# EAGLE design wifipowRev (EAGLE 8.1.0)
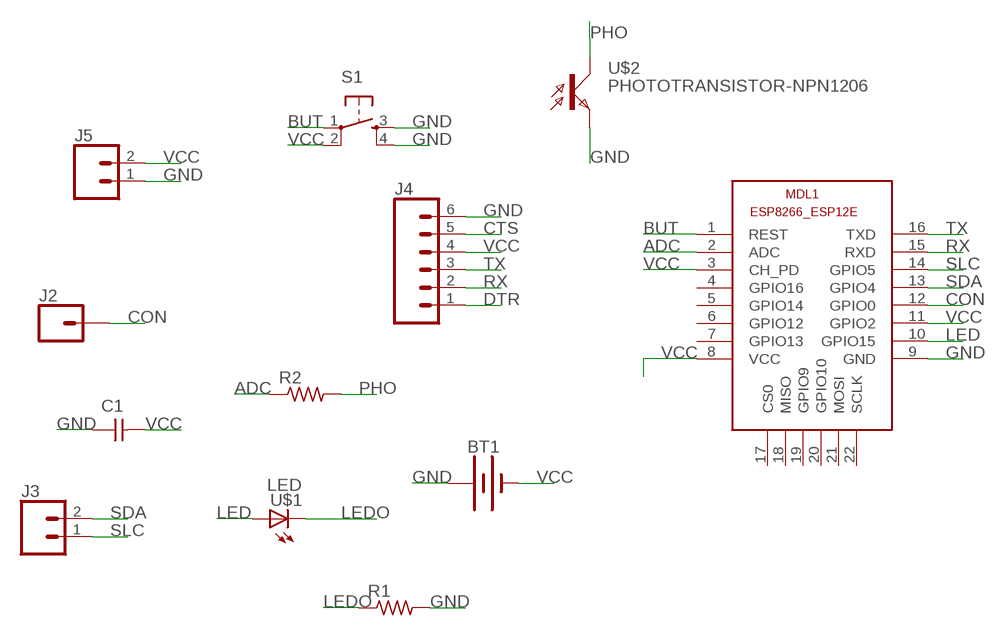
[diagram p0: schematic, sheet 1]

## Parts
BT1  BATTERY-20MM_SMD  [BATTCON_20MM]
C1  CAP-UNPOLARIZEDFAB  [C1206FAB]
J2  CONN_01PTH_LONGPAD  [1X01_LONGPAD]
J3  CONN_02PTH3  [1X02_LONGPADS]
J4  CONN_06LONGPADS  [1X06_LONGPADS]
J5  CONN_02PTH3  [1X02_LONGPADS]
MDL1  ESP8266-12EESP8266-ESP12E  [ESP8266-ESP12E]
R1  RES-US1206  [R1206]
R2  RES-US1206FAB  [R1206FAB]
S1  6MM_SWITCH6MM_SWITCH  [6MM_SWITCH]
U$1  LED  [LED1206]
U$2  PHOTOTRANSISTOR-NPN1206  [OP1206]

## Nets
ADC: MDL1.2(ADC) R2.1
BUT: MDL1.1(REST) S1.1(P)
CON: J2.1 MDL1.12(GPIO0)
CTS: J4.5
DTR: J4.1
GND: BT1.1(+) C1.1 J4.6 J5.1 MDL1.9(GND) R1.2 S1.3(S) S1.4(S1) U$2.EMITTER(E)
LED: MDL1.10(GPIO15) U$1.1(A)
LEDO: R1.1 U$1.2(C)
PHO: R2.2 U$2.COLLECTOR(C)
RX: J4.2 MDL1.15(RXD)
SDA: J3.2 MDL1.13(GPIO4)
SLC: J3.1 MDL1.14(GPIO5)
TX: J4.3 MDL1.16(TXD)
VCC: BT1.2(-) C1.2 J4.4 J5.2 MDL1.3(CH_PD) MDL1.8(VCC) MDL1.11(GPIO2) S1.2(P1)
Unconnected: MDL1.4(GPIO16) MDL1.5(GPIO14) MDL1.6(GPIO12) MDL1.7(GPIO13) MDL1.17(CS0) MDL1.18(MISO) MDL1.19(GPIO9) MDL1.20(GPIO10) MDL1.21(MOSI) MDL1.22(SCLK)

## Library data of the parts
BT1 = SparkFun-Batteries:BATTERY: Battery - Single Cell; PROD_ID: BATT-11519
C1 = fab:CAP-UNPOLARIZED
J2 = SparkFun-Connectors:CONN_01: Single connection point. Often used as Generic Header-pin footprint for 0.1 inch spaced/style header connections
J3 J5 = SparkFun-Connectors:CONN_02: Multi connection point. Often used as Generic Header-pin footprint for 0.1 inch spaced/style header connections
J4 = SparkFun-Connectors:CONN_06: Multi connection point. Often used as Generic Header-pin footprint for 0.1 inch spaced/style header connections On any of the 0.1 inch spaced packages, you can populate with these: Break Away Headers - Straight (PRT-00116) Break Away Male Headers - Right Angle (PRT-00553) Female Headers (PRT-00115)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
MDL1 = ESP8266-ESP12E:ESP8266-12E: ESP8266-12E with additional I/O and GPIO04/05 corrected The author cannot warrant that this library is free from error or will meet your specific requirements. Created by PuceBaboon.com. Komagane, Nagano, JAPAN
R1 R2 = fab:RES-US: Resistor (US Symbol)
S1 = fab:6MM_SWITCH: OMRON SWITCH
U$1 = fab:LED: LED
U$2 = fab:PHOTOTRANSISTOR-NPN

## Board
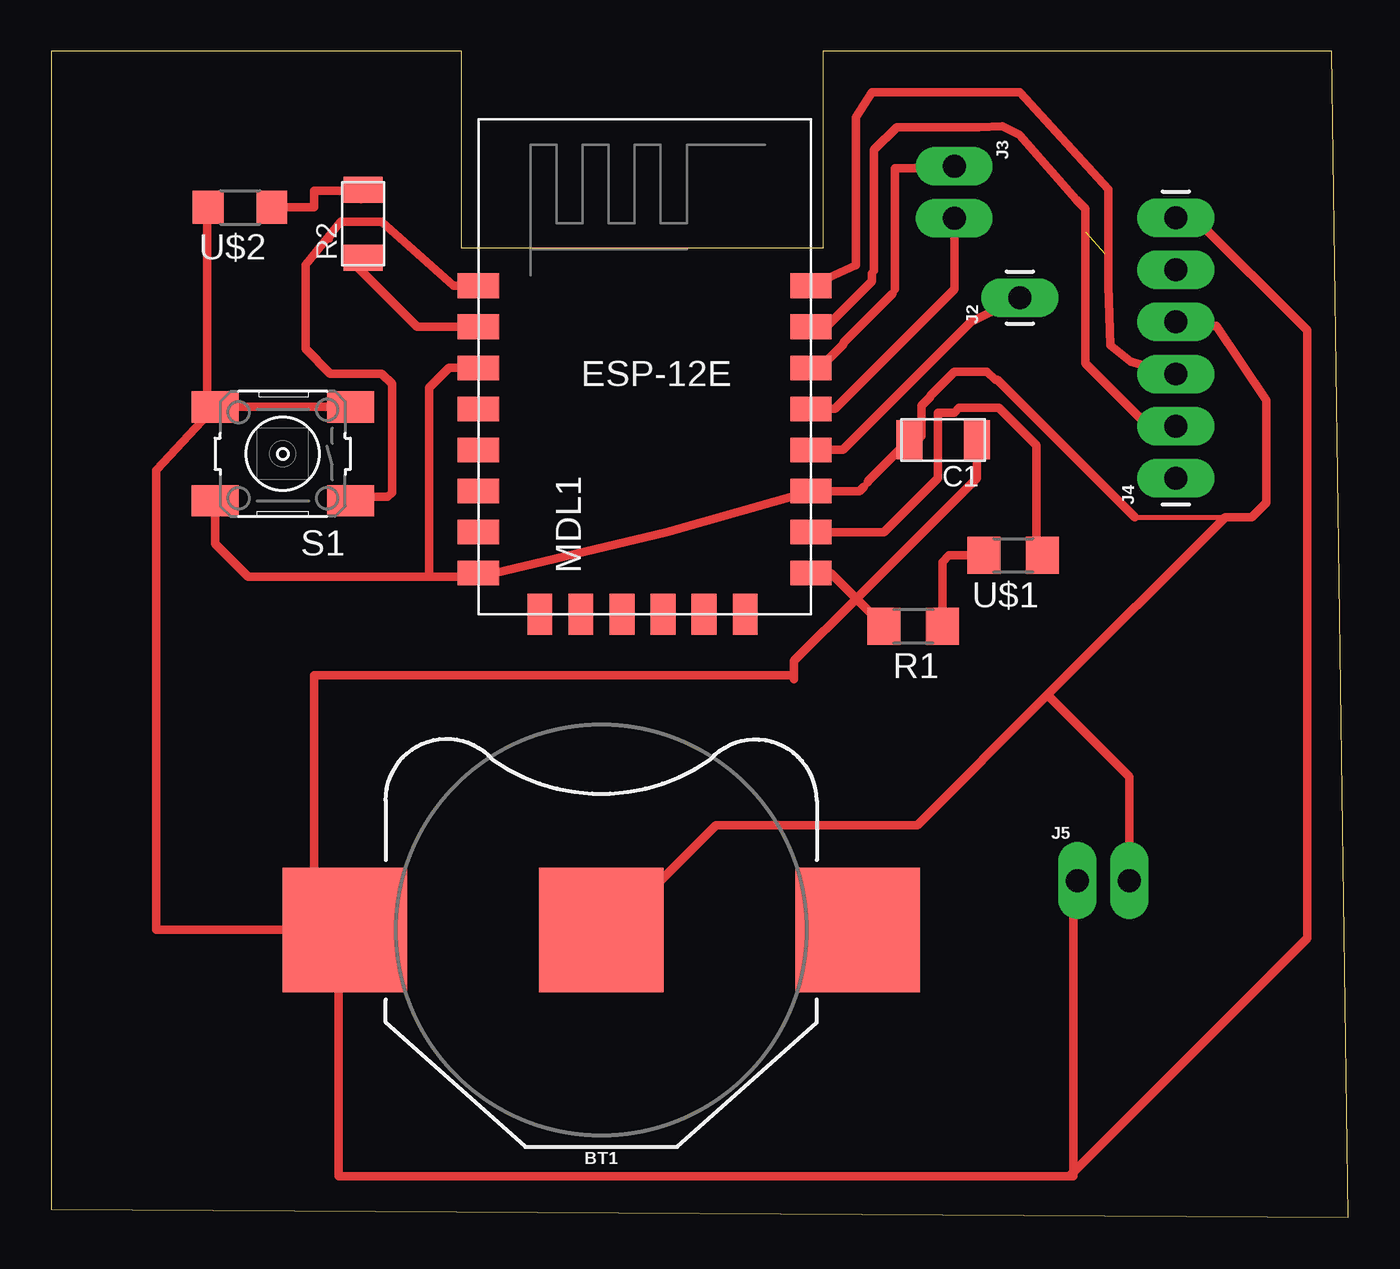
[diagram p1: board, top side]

Size 63.2 x 56.8 mm. Coordinates in mm from the lower left corner, seen from the top.
Outline: 0,0.4 63.2,0 62.4,56.8 37.6,56.8 37.6,47.2 20,47.2 20,56.8 0,56.8 0,0.4
Copper layers (1*16): Top 0.035mm / dielectric 1.5mm / Bottom 0.035mm
Design rules "default *": minimum track width 10mil, minimum drill 24mil, track to track 0.4mm, track to pad 0.4mm, pad to pad 0.4mm, via to via 0.4mm, smd to smd 0.4mm, copper to edge 40mil, drill to drill 8mil, minimum pad ring 10mil, minimum via ring 8mil, stop-mask expansion 4mil, vias tented up to drill 0mil, thermal gap 10mil

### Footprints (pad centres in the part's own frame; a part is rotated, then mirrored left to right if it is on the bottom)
BATTCON_20MM = smd 6.07 x 6.07: 1 -12.5,0; 2 0,0; 3 12.5,0
C1206FAB = smd 1.27 x 1.905: 1 -1.651,0; 2 1.651,0
1X01_LONGPAD = drill 1.118 pad 1.88 long: 1 0,0
1X02_LONGPADS = drill 1.118 pad 1.88 long: 1 0,0; 2 2.54,0
1X06_LONGPADS = drill 1.118 pad 1.88 long: 1 0,0; 2 2.54,0; 3 5.08,0; 4 7.62,0; 5 10.16,0; 6 12.7,0
ESP8266-ESP12E = smd 2 x 1.2: 1 -7.62,5.84; 2 -7.62,3.84; 3 -7.62,1.84; 4 -7.62,-0.16; 5 -7.62,-2.16; 6 -7.62,-4.16; 7 -7.62,-6.16; 8 -7.62,-8.16; 9 8.58,-8.16; 10 8.58,-6.16; 11 8.58,-4.16; 12 8.58,-2.16; 13 8.58,-0.16; 14 8.58,1.84; 15 8.58,3.84; 16 8.58,5.84 | smd 1.2 x 2: 17 -4.62,-10.16; 18 -2.62,-10.16; 19 -0.62,-10.16; 20 1.38,-10.16; 21 3.38,-10.16; 22 5.38,-10.16
R1206 = smd 1.6 x 1.803: 1 -1.422,0; 2 1.422,0
R1206FAB = smd 1.27 x 1.905: 1 -1.651,0; 2 1.651,0
6MM_SWITCH = smd 2.286 x 1.524: 1 -3.302,2.286; 2 3.302,2.286; 3 -3.302,-2.286; 4 3.302,-2.286
LED1206 = smd 1.6 x 1.803: 1 -1.422,0; 2 1.422,0
OP1206 = smd 1.5 x 1.6: COLLECTOR -1.55,0; EMITTER 1.55,0

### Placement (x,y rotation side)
BT1  26.8,14 0 top
C1  43.46,37.87 180 top
J2  47.2,44.8 90 top
J3  44,51.2 270 top
J4  54.8,36 90 top
J5  50,16.4 0 top
MDL1  28.43,39.54 0 top
R1  42,28.8 180 top
R2  15.2,48.4 90 top
S1  11.28,37.19 180 top
U$1  46.87,32.25 180 top
U$2  9.2,49.2 180 top

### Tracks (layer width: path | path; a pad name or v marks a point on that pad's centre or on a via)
ADC
  Top 0.254: R2.1 15.6,46.6 | 20.6,43.6 MDL1.2
  Top 0.406: MDL1.2 17.82,43.38 14.8,46.4 14.85,46.4 R2.1
BUT
  Top 0.254: 13.6,47.6 14.1,48.5
  Top 0.406: MDL1.1 19.61,45.39 16.1,48.5 14.1,48.5 12.4,46.4 12.4,42.3 13.6,41.1 16.1,41.1 16.6,40.6 16.6,35.3 16.4,35.1 14.78,35.1 S1.1 14.58,34.58 14.4,34.4 14,34.8
CON
  Top 0.254: 37.1,37.6 MDL1.12
  Top 0.406: MDL1.12 38.58,37.38 44.8,43.6 J2.1
GND
  Top 0.254: 7.6,48.8 7.6,49.1 U$2.EMITTER | 14.1,39.6 S1.3 | 45.1,37.2 45.1,37.6 C1.1 | 16.6,11.6 14.6,13.6 BT1.1 | 49.81,16.26 J5.1
  Top 0.406: BT1.1 12.8,14 12.8,26.4 36.2,26.4 | 36.2,26.4 36.2,26.2 | BT1.1 14,14 14,2 49.6,2 | 49.6,2 49.81,2 49.81,16.26 | BT1.1 5.1,14 5.1,36.4 S1.4 | S1.4 7.6,39.48 7.6,48.8 | S1.4 14.1,39.48 14.1,39.6 | 54.4,49.1 J4.6 55.7,48.7 61.2,43.2 61.2,13.6 49.6,2 | 39.24,30.14 36.2,27.1 36.2,26.4 | 39.24,30.14 45.1,36 45.1,37.2 | 45.1,37.2 45.1,38.3 45.2,38.4 45.2,37.3 45.1,37.2 | 39.24,30.14 R1.2 | MDL1.9 38,31.38 39.24,30.14
LED
  Top 0.406: MDL1.10 40.58,33.38 43.2,36 43.2,39.2 44,39.2 44.23,39.43 46.17,39.43 48,37.6 48,32.54 U$1.1
LEDO
  Top 0.406: R1.1 43.42,31.92 43.75,32.25 U$1.2
PHO
  Top 0.254: 11.1,49.6 U$2.COLLECTOR | 15.1,49.6 R2.2
  Top 0.406: U$2.COLLECTOR 12.8,49.2 12.8,50 15.1,50 15.1,49.6
RX  (1 unrouted)
  Top 0.254: 40.1,46.1 40,46
  Top 0.406: J4.2 53.46,38.54 50.4,41.6 50.4,48 50.4,49.12 49.96,49.56 47.18,52.74 46.36,53.14 45.2,53.1 41.2,53.1 40.1,52 40.1,46.1 | 40,46 40,45.6 37.6,43.2 37.19,43.2 MDL1.15
SDA
  Top 0.406: MDL1.13 38.18,39.38 44,45.2 J3.2
SLC
  Top 0.254: 41,45 41.1,45.1 41.1,45.2 | 41.1,51.1 41.2,51.1
  Top 0.406: 41,45 38.61,42.61 38.61,42.53 37.46,41.38 MDL1.14 | 41.1,45.2 41.1,51.1 | 41.2,51.1 43.9,51.1 J3.1
TX
  Top 0.406: J4.3 52.6,41.68 51.62,42.48 51.52,45.38 51.52,50.08 47.2,54.8 40,54.8 39.2,53.6 39.2,46.37 MDL1.16
VCC  (1 unrouted)
  Top 0.254: 39.6,35.6 39.8,35.8 | 20.6,41.1 MDL1.3 | 52.1,16.6 J5.2 | 55.1,43.6 J4.4 | 52.8,34.1 57.2,34.1
  Top 0.406: S1.2 7.98,32.82 9.6,31.2 18.4,31.2 | 18.4,31.2 20.63,31.2 MDL1.8 21.58,31.38 29.98,33.38 MDL1.11 39.38,35.38 39.6,35.6 | MDL1.3 19.38,41.38 18.4,40.4 18.4,31.2 | BT1.2 27.3,14 32.4,19.1 42.2,19.1 48.55,25.45 | 48.55,25.45 57.2,34.1 58.5,34.1 59.2,34.8 59.2,39.8 56.78,43.42 56.48,43.42 55.1,43.6 | J5.2 52.54,21.46 48.55,25.45 | 52.8,34.1 46.1,40.8 46,40.8 45.6,41.2 44,41.2 42.83,40.03 42.83,39.97 42.39,39.53 42.39,38.05 42.21,37.87 C1.2 39.8,35.86 39.8,35.8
